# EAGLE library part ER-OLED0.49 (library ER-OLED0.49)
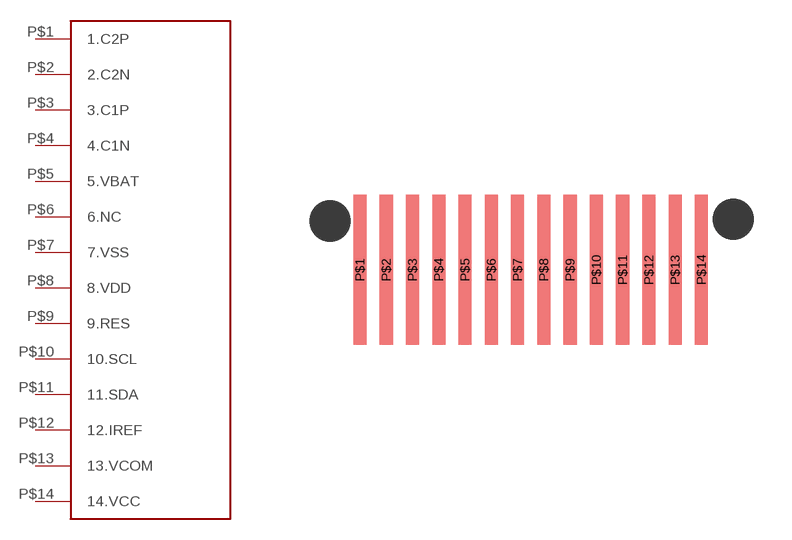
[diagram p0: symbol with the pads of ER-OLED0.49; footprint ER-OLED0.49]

Designator prefix -

## ER-OLED0.49  [ER-OLED0.49]
P$1  1.C2P
P$2  2.C2N
P$3  3.C1P
P$4  4.C1N
P$5  5.VBAT
P$6  6.NC
P$7  7.VSS
P$8  8.VDD
P$9  9.RES
P$10  10.SCL
P$11  11.SDA
P$12  12.IREF
P$13  13.VCOM
P$14  14.VCC

## Footprint ER-OLED0.49 (pad centres in mm)
smd 0.35 x 4: P$1 1.45,2; P$2 2.15,2; P$3 2.85,2; P$4 3.55,2; P$5 4.25,2; P$6 4.95,2; P$7 5.65,2; P$8 6.35,2; P$9 7.05,2; P$10 7.75,2; P$11 8.45,2; P$12 9.15,2; P$13 9.85,2; P$14 10.55,2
